(* 使用CoE驱动器内部回零模式进行回零 *)
FUNCTION_BLOCK FB_DiverBasedHoming
VAR_IN_OUT
	AxisRef		: AXIS_REF;		(* PLC轴对象 *)
END_VAR
VAR_INPUT
	bExcute		: BOOL;(* 上升沿触发回零动作 *)
	bReset		: BOOL;(* 上升沿复位回零错误 *)
	stParameter	: ST_Parameter_HomeParaCoE;(* 驱动器回零参数 *) 
END_VAR
VAR_OUTPUT
	bHoming						: BOOL;(* 回零中 *)
	bError						: BOOL;(* 错误 *)
	nErrorID					: UDINT;(* 错误号 *)
	eHomeStep					: E_DriverHomeStep := STATE_DRIVERHOME_DONE;(* 回零状态机 *)
END_VAR
VAR
	fbChangeMode				: MC_WriteDriveOperationMode;
	fbWriteNcIoOutput			: MC_WriteNcIoOutput;
	fbWriteCoEHomeMethod		: FB_CoEWrite;
	fbWriteCoEHomeAcceleration	: FB_CoEWrite;
	fbWriteCoEVelocityForSwitch	: FB_CoEWrite;
	fbWriteCoEVelocityForIndex	: FB_CoEWrite;
	fbWriteCoEHomeOffset		: FB_CoEWrite;	
	fbReadParameter				: MC_ReadParameter;
	fbReadStatusWord			: FB_CoERead;	
	fbReset						: MC_Reset;
	fbWriteBoolParameter		: MC_WriteBoolParameter;
	fbSetPosition				: MC_SetPosition;
	fbHome						: MC_Home;
	
	HomeMethod					: SINT;
	Acceleration				: UDINT;
	VelocityForSwitch			: UDINT;
	VelocityForIndex			: UDINT;
	HomeOffset					: DINT;
	fScalingFactor				: LREAL;
	StatusWord					: UINT;
	
	bHomeDone					: BOOL;
	bHomeError					: BOOL;
	
	fbTonReadStatus				: TON;
	nPositionActualValue		: DINT;
	nTest						: UINT;
	rtExecute					: R_TRIG;
	rtReset						: R_TRIG;
	
END_VAR

rtExecute( CLK := bExcute );
rtReset( CLK := bReset );
IF rtExecute.Q = TRUE THEN(* 执行命令触发时，清空所有功能块输入 *)
	fbHome						.Execute	:= FALSE;
	fbWriteNcIoOutput			.Execute	:= FALSE;
	fbChangeMode				.Execute	:= FALSE;
	fbWriteCoEHomeMethod		.Execute	:= FALSE;
	fbWriteCoEHomeAcceleration	.Execute	:= FALSE;
	fbWriteCoEVelocityForSwitch	.Execute	:= FALSE;
	fbWriteCoEVelocityForIndex	.Execute	:= FALSE;
	fbWriteCoEHomeOffset		.Execute	:= FALSE;
	fbReadParameter				.Enable		:= FALSE;
	fbReadStatusWord			.Execute	:= FALSE;
	fbTonReadStatus				.IN			:= FALSE;
	fbReset						.Execute	:= FALSE;
	fbWriteBoolParameter		.Execute	:= FALSE;
	fbSetPosition				.Execute	:= FALSE;
	eHomeStep	:= STATE_DRIVERHOME_CLEARFLAG;
ELSIF rtReset.Q = TRUE THEN(* 复位命令触发时，清空所有功能块输入 *)
	fbWriteNcIoOutput			.Execute	:= FALSE;
	fbChangeMode				.Execute	:= FALSE;
	fbWriteCoEHomeMethod		.Execute	:= FALSE;
	fbWriteCoEHomeAcceleration	.Execute	:= FALSE;
	fbWriteCoEVelocityForSwitch	.Execute	:= FALSE;
	fbWriteCoEVelocityForIndex	.Execute	:= FALSE;
	fbWriteCoEHomeOffset		.Execute	:= FALSE;
	fbReadParameter				.Enable		:= FALSE;
	fbReadStatusWord			.Execute	:= FALSE;
	fbTonReadStatus				.IN			:= FALSE;
	fbReset						.Execute	:= FALSE;
	fbWriteBoolParameter		.Execute	:= FALSE;
	fbSetPosition				.Execute	:= FALSE;
	IF eHomeStep = STATE_DRIVERHOME_ERROR THEN
		eHomeStep	:= STATE_DRIVERHOME_STOP2;
	ELSE
		eHomeStep	:= STATE_DRIVERHOME_STOP1;
	END_IF
	bError := FALSE;
	nErrorID	:= 0;
END_IF

(* 显示回零中状态 *)
bHoming	:= FALSE;
IF eHomeStep >= STATE_DRIVERHOME_CLEARFLAG AND eHomeStep <= STATE_DRIVERHOME_SET_FLAG THEN
	bHoming	:= TRUE;
END_IF

(* 错误发生时，强制跳转进入错误停止，发送停止控制字 *)
IF ( AxisRef.Status.Error = TRUE ) AND eHomeStep > STATE_DRIVERHOME_STANDSTILL AND eHomeStep < STATE_DRIVERHOME_ERRORSTOP THEN
	eHomeStep := STATE_DRIVERHOME_ERRORSTOP;
END_IF


(* 状态机逻辑 *)
CASE eHomeStep OF
STATE_DRIVERHOME_STANDSTILL:(* 待命，可以触发回零命令 *)
	;
(* ------------------------- 回零逻辑 ---------------------------- *)
STATE_DRIVERHOME_CLEARFLAG:(* 清除回零标志 *)
	fbHome.HomingMode		:= MC_HomingMode.MC_ResetCalibration;
	fbHome.Execute			:= TRUE;
	IF fbHome.Done THEN
		fbHome.Execute		:= FALSE;
		eHomeStep 			:= STATE_DRIVERHOME_DISABLELAG;
	ELSIF fbHome.Error THEN
		fbHome.Execute		:= FALSE;
		eHomeStep 			:= STATE_DRIVERHOME_ERRORSTOP;
	END_IF
	
STATE_DRIVERHOME_DISABLELAG:(* 禁用跟随误差监控 *)
	fbWriteBoolParameter.Value := FALSE;
	fbWriteBoolParameter.ParameterNumber := MC_AxisParameter.EnablePosLagMonitoring;
	fbWriteBoolParameter.Execute	:= TRUE;
	IF fbWriteBoolParameter.Done = TRUE THEN
		fbWriteBoolParameter.Execute	:= FALSE;
		eHomeStep := STATE_DRIVERHOME_READSCLFCTR;
	END_IF
	IF fbWriteBoolParameter.Error = TRUE THEN
		fbWriteBoolParameter.Execute	:= FALSE;
		nErrorID := fbWriteBoolParameter.ErrorID;
		eHomeStep := STATE_DRIVERHOME_ERRORSTOP;
	END_IF
	
STATE_DRIVERHOME_READSCLFCTR:(* 读取编码器 齿轮比系数 *)
	fbReadParameter.ParameterNumber := MC_AxisParameter.AxisEncoderScalingFactor;
	fbReadParameter.ReadMode		:= E_ReadMode.READMODE_ONCE;
	fbReadParameter.Enable		:=	TRUE;
	IF fbReadParameter.Valid THEN
		fbReadParameter.Enable		:=	FALSE;
		fScalingFactor := fbReadParameter.Value;
		HomeMethod 			:= stParameter.HomeMethod;
		Acceleration 		:= LREAL_TO_UDINT(stParameter.Acceleration / fScalingFactor) ;
		VelocityForSwitch 	:= LREAL_TO_UDINT(stParameter.VelocityForSwitch / fScalingFactor) ;
		VelocityForIndex	:= LREAL_TO_UDINT(stParameter.VelocityForIndex / fScalingFactor) ;
		HomeOffset			:= LREAL_TO_DINT(stParameter.HomeOffset / fScalingFactor) ;
		eHomeStep := STATE_DRIVERHOME_MODEHOME;
	END_IF
	IF fbReadParameter.Error = TRUE THEN
		fbReadParameter.Enable	:= FALSE;
		nErrorID := fbReadParameter.ErrorID;
		eHomeStep := STATE_DRIVERHOME_ERRORSTOP;
	END_IF
	
STATE_DRIVERHOME_MODEHOME:(* 切换到回零模式 *)
	fbChangeMode.DriveOperationMode := E_DriveOperationMode.DriveOperationMode_DriveBasedHoming;
	fbChangeMode.Execute			:= TRUE;
	IF fbChangeMode.Done THEN
		fbChangeMode.Execute			:= FALSE;
		eHomeStep 			:= STATE_DRIVERHOME_WRITEPARA1;
	END_IF
	IF fbChangeMode.Error = TRUE THEN
		fbChangeMode.Execute	:= FALSE;
		nErrorID := fbChangeMode.ErrorID;
		eHomeStep := STATE_DRIVERHOME_ERRORSTOP;
	END_IF
	
STATE_DRIVERHOME_WRITEPARA1:(* 写入回零参数到驱动器 *)
	fbWriteCoEHomeMethod.Index		:= 16#6098;
	fbWriteCoEHomeMethod.SubIndex	:= 0;
	fbWriteCoEHomeMethod.pSrcBuf	:= ADR( HomeMethod );
	fbWriteCoEHomeMethod.BufLen		:= SIZEOF( HomeMethod );
	fbWriteCoEHomeMethod.Execute	:= TRUE;
	
	fbWriteCoEVelocityForSwitch.Index	:= 16#6099;
	fbWriteCoEVelocityForSwitch.SubIndex:= 1;
	fbWriteCoEVelocityForSwitch.pSrcBuf	:= ADR( VelocityForSwitch );
	fbWriteCoEVelocityForSwitch.BufLen	:= SIZEOF( VelocityForSwitch );
	fbWriteCoEVelocityForSwitch.Execute	:= TRUE;
	
	fbWriteCoEVelocityForIndex.Index	:= 16#6099;
	fbWriteCoEVelocityForIndex.SubIndex	:= 2;
	fbWriteCoEVelocityForIndex.pSrcBuf	:= ADR( VelocityForIndex );
	fbWriteCoEVelocityForIndex.BufLen	:= SIZEOF( VelocityForIndex );
	fbWriteCoEVelocityForIndex.Execute	:= TRUE;
	
	fbWriteCoEHomeOffset.Index		:= 16#607C;
	fbWriteCoEHomeOffset.SubIndex	:= 0;
	fbWriteCoEHomeOffset.pSrcBuf	:= ADR( HomeOffset );
	fbWriteCoEHomeOffset.BufLen		:= SIZEOF( HomeOffset );
	fbWriteCoEHomeOffset.Execute	:= TRUE;
	
	fbWriteCoEHomeAcceleration.Index		:= 16#609A;
	fbWriteCoEHomeAcceleration.SubIndex	:= 0;
	fbWriteCoEHomeAcceleration.pSrcBuf	:= ADR( Acceleration );
	fbWriteCoEHomeAcceleration.BufLen		:= SIZEOF( Acceleration );
	fbWriteCoEHomeAcceleration.Execute	:= TRUE;
	
	eHomeStep 			:= STATE_DRIVERHOME_WRITEPARA2;	
	
STATE_DRIVERHOME_WRITEPARA2:(* 等待参数写入完成 *)
	IF 	fbWriteCoEHomeMethod.Busy = FALSE 
		AND fbWriteCoEVelocityForSwitch.Busy = FALSE
		AND fbWriteCoEVelocityForIndex.Busy = FALSE
		AND fbWriteCoEHomeOffset.Busy = FALSE 
		AND fbWriteCoEHomeAcceleration.Busy = FALSE THEN
		fbWriteCoEHomeMethod.Execute		:= FALSE;
		fbWriteCoEVelocityForSwitch.Execute	:= FALSE;
		fbWriteCoEVelocityForIndex.Execute	:= FALSE;
		fbWriteCoEHomeOffset.Execute		:= FALSE;
		fbWriteCoEHomeAcceleration.Execute	:= FALSE;
		eHomeStep 			:= STATE_DRIVERHOME_STARTHOME;
	END_IF
	IF 	fbWriteCoEHomeMethod.Error = TRUE 
		OR fbWriteCoEVelocityForSwitch.Error = TRUE
		OR fbWriteCoEVelocityForIndex.Error = TRUE
		OR fbWriteCoEHomeOffset.Error 		= TRUE 
		OR fbWriteCoEHomeAcceleration.Error = TRUE THEN
		
		fbWriteCoEHomeMethod.Execute		:= FALSE;
		fbWriteCoEVelocityForSwitch.Execute	:= FALSE;
		fbWriteCoEVelocityForIndex.Execute	:= FALSE;
		fbWriteCoEHomeOffset.Execute		:= FALSE;
		fbWriteCoEHomeAcceleration.Execute	:= FALSE;
		
		nErrorID	:= fbWriteCoEHomeMethod.AdsErrId
						OR fbWriteCoEVelocityForSwitch.AdsErrId 
						OR fbWriteCoEVelocityForIndex.AdsErrId
						OR fbWriteCoEHomeOffset.AdsErrId 		
						OR fbWriteCoEHomeAcceleration.AdsErrId ;
		eHomeStep 			:= STATE_DRIVERHOME_ERRORSTOP;
	END_IF	
		
STATE_DRIVERHOME_STARTHOME:(* 写控制字触发驱动器回零 *)
	fbWriteNcIoOutput.Device 		:= E_NcIoDevice.NcIoDeviceDrive;
	fbWriteNcIoOutput.NcIoOutput	:= E_NcIoOutput.NcIoOutputnCtrl1;
	fbWriteNcIoOutput.BitSelectMask	:= 16#110;
	fbWriteNcIoOutput.BitValues    	:= 16#10;
	fbWriteNcIoOutput.Execute		:= TRUE;
	IF fbWriteNcIoOutput.Done THEN
		fbWriteNcIoOutput.Execute		:= FALSE;
		StatusWord := 0;
		bHomeError := 0;
		bHomeDone	:= 0;
		eHomeStep 			:= STATE_DRIVERHOME_CHECKSTATUS1;
	END_IF
	IF fbWriteNcIoOutput.Error = TRUE THEN
		fbWriteNcIoOutput.Execute	:= FALSE;
		nErrorID := fbWriteNcIoOutput.ErrorID;
		eHomeStep := STATE_DRIVERHOME_ERRORSTOP;
	END_IF
	
STATE_DRIVERHOME_CHECKSTATUS1:(* 使用SDO读状态字 *)
	fbReadStatusWord.Index 		:= 16#6041;
	fbReadStatusWord.SubIndex 	:= 0;
	fbReadStatusWord.pDstBuf	:= ADR(StatusWord);
	fbReadStatusWord.BufLen		:= SIZEOF(StatusWord);
	fbReadStatusWord.Execute	:= TRUE;
	eHomeStep 			:= STATE_DRIVERHOME_CHECKSTATUS2;
	
STATE_DRIVERHOME_CHECKSTATUS2:(* 检查状态字中的回零完成和回零错误位 *)
	IF fbReadStatusWord.Busy = FALSE THEN
		fbReadStatusWord.Execute	:= FALSE;
		bHomeError 	:= StatusWord.13;
		bHomeDone 	:= StatusWord.12;
		IF bHomeError = TRUE THEN(* 回零错误进入错误状态机 *)
			nErrorID			:= 666;
			eHomeStep 			:= STATE_DRIVERHOME_ERRORSTOP;
		ELSIF bHomeDone = TRUE THEN(* 回零完成 *)
			eHomeStep 			:= STATE_DRIVERHOME_RESETSETPOINT;
		ELSE
			fbTonReadStatus.IN := TRUE;
		END_IF
	END_IF
	
	IF fbTonReadStatus.Q THEN(* 返回循环读取检查状态 *)
		fbTonReadStatus.IN := FALSE;
		eHomeStep 			:= STATE_DRIVERHOME_CHECKSTATUS1;
	END_IF
	
	IF fbReadStatusWord.Error = TRUE THEN
		fbReadStatusWord.Execute	:= FALSE;
		fbTonReadStatus.IN := FALSE;
		nErrorID := fbReadStatusWord.AdsErrId;
		eHomeStep := STATE_DRIVERHOME_ERRORSTOP;
	END_IF
	
STATE_DRIVERHOME_RESETSETPOINT:(* 回零完成后触发复位命令，目的是切换到CSP之前使设定位置和当前位置一致 *)
	fbReset.Execute := TRUE;
	IF 	fbReset.Done THEN
		fbReset.Execute := FALSE;
		eHomeStep 			:= STATE_DRIVERHOME_MODECSP;
	END_IF
	IF 	fbReset.Error THEN
		fbReset.Execute := FALSE;
		nErrorID := fbReset.ErrorID;
		eHomeStep 			:= STATE_DRIVERHOME_ERRORSTOP;
	END_IF
STATE_DRIVERHOME_MODECSP:(* 切换回CSP模式 *)
	fbChangeMode.DriveOperationMode := E_DriveOperationMode.DriveOperationMode_Pos1;
	fbChangeMode.Execute			:= TRUE;
	IF fbChangeMode.Done THEN
		fbChangeMode.Execute			:= FALSE;
		(* 切换回CSP模式后读取驱动器显示的当前位置 *)
		fbReadStatusWord.Index 		:= 16#6064;
		fbReadStatusWord.SubIndex 	:= 0;
		fbReadStatusWord.pDstBuf	:= ADR(nPositionActualValue);
		fbReadStatusWord.BufLen		:= SIZEOF(nPositionActualValue);
		fbReadStatusWord.Execute	:= TRUE;
		
		eHomeStep 			:= STATE_DRIVERHOME_READPOSITION;
	END_IF
	IF fbChangeMode.Error = TRUE THEN
		fbChangeMode.Execute	:= FALSE;
		nErrorID := fbChangeMode.ErrorID;
		eHomeStep := STATE_DRIVERHOME_ERRORSTOP;
	END_IF
	
STATE_DRIVERHOME_READPOSITION:(* 读取驱动器显示的当前位置 完成 *)
	IF fbReadStatusWord.Busy = FALSE THEN
		eHomeStep 			:= STATE_DRIVERHOME_CLEARPOS;
	END_IF
	IF fbReadStatusWord.Error = TRUE THEN
		fbReadStatusWord.Execute	:= FALSE;
		nErrorID := fbReadStatusWord.AdsErrId;
		eHomeStep := STATE_DRIVERHOME_ERRORSTOP;
	END_IF
	
STATE_DRIVERHOME_CLEARPOS:(* 用驱动器反馈的位置替换NC显示的位置 *)
	fbSetPosition.Position	:= nPositionActualValue * fScalingFactor;
	fbSetPosition.Execute 	:= TRUE;
	IF fbSetPosition.Done = TRUE THEN
		fbSetPosition.Execute 	:= FALSE;
		eHomeStep 			:= STATE_DRIVERHOME_ENABLELAG;
	END_IF
	IF fbSetPosition.Error = TRUE THEN
		fbSetPosition.Execute	:= FALSE;
		nErrorID := fbSetPosition.ErrorID;
		eHomeStep := STATE_DRIVERHOME_ERRORSTOP;
	END_IF
	
STATE_DRIVERHOME_ENABLELAG:(* 启用跟随误差监控 *)
	fbWriteBoolParameter.Value := TRUE;
	fbWriteBoolParameter.ParameterNumber := MC_AxisParameter.EnablePosLagMonitoring;
	fbWriteBoolParameter.Execute	:= TRUE;
	IF fbWriteBoolParameter.Done = TRUE THEN
		fbWriteBoolParameter.Execute	:= FALSE;
		eHomeStep := STATE_DRIVERHOME_SET_FLAG; (* 进入回零完成状态机 *)
	END_IF
	IF fbWriteBoolParameter.Error = TRUE THEN
		fbWriteBoolParameter.Execute	:= FALSE;
		nErrorID := fbWriteBoolParameter.ErrorID;
		eHomeStep := STATE_DRIVERHOME_ERRORSTOP;
	END_IF
	
STATE_DRIVERHOME_SET_FLAG:(* 设置回零标志 *)
	fbHome.HomingMode		:= MC_HomingMode.MC_ForceCalibration;
	fbHome.Execute			:= TRUE;
	IF fbHome.Done THEN
		fbHome.Execute		:= FALSE;
		eHomeStep 			:= STATE_DRIVERHOME_DONE;
	ELSIF fbHome.Error THEN
		fbHome.Execute		:= FALSE;
		eHomeStep 			:= STATE_DRIVERHOME_ERRORSTOP;
	END_IF
	
	
(* ------------------------- 复位逻辑 ---------------------------- *)
STATE_DRIVERHOME_STOP1:(* 发送 停止控制字 *)
	fbWriteNcIoOutput.Device 		:= E_NcIoDevice.NcIoDeviceDrive;
	fbWriteNcIoOutput.NcIoOutput	:= E_NcIoOutput.NcIoOutputnCtrl1;
	fbWriteNcIoOutput.BitSelectMask	:= 16#110;
	fbWriteNcIoOutput.BitValues    	:= 16#100;
	fbWriteNcIoOutput.Execute		:= TRUE;
	IF fbWriteNcIoOutput.Done THEN
		fbWriteNcIoOutput.Execute		:= FALSE;
		StatusWord := 0;
		bHomeError := 0;
		bHomeDone	:= 0;
		
		eHomeStep 			:= STATE_DRIVERHOME_STOP2;
	END_IF
STATE_DRIVERHOME_STOP2:(* 延时后复位该控制字*)
	fbTonReadStatus.IN := TRUE;
	IF 	fbTonReadStatus.Q THEN
		fbWriteNcIoOutput.Device 		:= E_NcIoDevice.NcIoDeviceDrive;
		fbWriteNcIoOutput.NcIoOutput	:= E_NcIoOutput.NcIoOutputnCtrl1;
		fbWriteNcIoOutput.BitSelectMask	:= 16#110;
		fbWriteNcIoOutput.BitValues    	:= 16#000;
		fbWriteNcIoOutput.Execute		:= TRUE;
		IF fbWriteNcIoOutput.Done THEN
			fbWriteNcIoOutput.Execute		:= FALSE;
			fbTonReadStatus.IN := FALSE;
			eHomeStep 			:= STATE_DRIVERHOME_STOP3;
		END_IF
	END_IF
	
STATE_DRIVERHOME_STOP3:(* 复位 以同步设定位置和当前位置 *)
	fbReset.Execute := TRUE;
	IF 	fbReset.Done THEN
		fbReset.Execute := FALSE;
		eHomeStep 			:= STATE_DRIVERHOME_STOP4;
	END_IF
	IF 	fbReset.Error THEN
		fbReset.Execute := FALSE;
		eHomeStep 			:= STATE_DRIVERHOME_STOP3;
	END_IF
	
STATE_DRIVERHOME_STOP4:(* 切换回CSP模式 *)
	fbChangeMode.DriveOperationMode := E_DriveOperationMode.DriveOperationMode_Pos1;
	fbChangeMode.Execute			:= TRUE;
	IF fbChangeMode.Done THEN
		fbChangeMode.Execute			:= FALSE;
		eHomeStep 			:= STATE_DRIVERHOME_STOP5;
	END_IF
	
STATE_DRIVERHOME_STOP5:(* 启用跟随误差监控 *)
	fbWriteBoolParameter.Value := TRUE;
	fbWriteBoolParameter.ParameterNumber := MC_AxisParameter.EnablePosLagMonitoring;
	fbWriteBoolParameter.Execute	:= TRUE;
	IF fbWriteBoolParameter.Done = TRUE THEN
		fbWriteBoolParameter.Execute	:= FALSE;
		eHomeStep := STATE_DRIVERHOME_STANDSTILL;
	END_IF
	
(* ------------------------- 出错逻辑 ---------------------------- *)	
STATE_DRIVERHOME_ERRORSTOP:(* 发送停止控制字 *)
	fbWriteNcIoOutput.Device 		:= E_NcIoDevice.NcIoDeviceDrive;
	fbWriteNcIoOutput.NcIoOutput	:= E_NcIoOutput.NcIoOutputnCtrl1;
	fbWriteNcIoOutput.BitSelectMask	:= 16#110;
	fbWriteNcIoOutput.BitValues    	:= 16#100;
	fbWriteNcIoOutput.Execute		:= TRUE;
	IF fbWriteNcIoOutput.Done THEN
		fbWriteNcIoOutput.Execute		:= FALSE;
		eHomeStep 			:= STATE_DRIVERHOME_ERROR;
	END_IF
	
STATE_DRIVERHOME_ERROR:(* 保留在错误状态机 *)
	bError := TRUE;	

END_CASE	

(* Call Function Blocks *)
fbWriteNcIoOutput			( Axis := AxisRef );
fbChangeMode				( Axis := AxisRef );
fbWriteCoEHomeMethod		( Axis := AxisRef );	
fbWriteCoEHomeAcceleration	( Axis := AxisRef );	
fbWriteCoEVelocityForSwitch	( Axis := AxisRef );
fbWriteCoEVelocityForIndex	( Axis := AxisRef );
fbWriteCoEHomeOffset		( Axis := AxisRef );	
fbReadParameter				( Axis := AxisRef );
fbReadStatusWord			( Axis := AxisRef );
fbTonReadStatus				( PT   := T#500MS );
fbReset						( Axis := AxisRef );
fbWriteBoolParameter		( Axis := AxisRef );
fbSetPosition				( Axis := AxisRef );

END_FUNCTION_BLOCK
